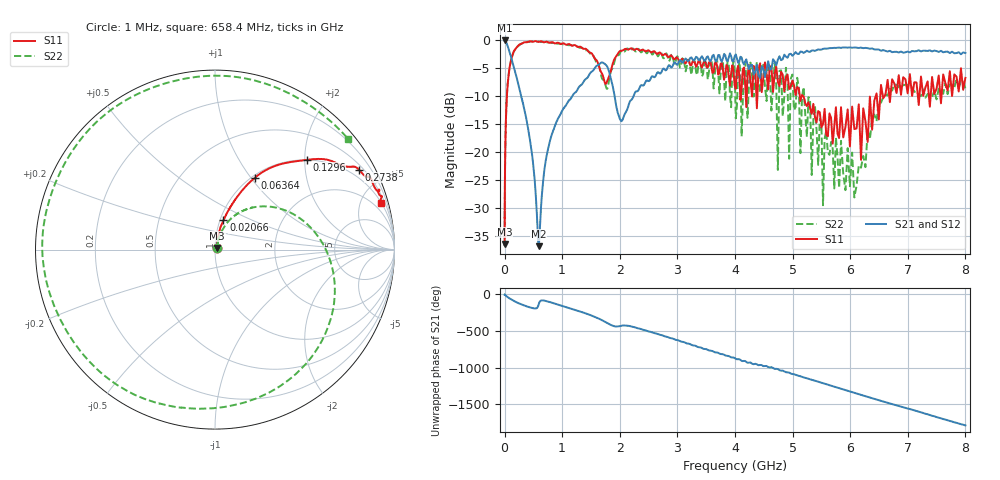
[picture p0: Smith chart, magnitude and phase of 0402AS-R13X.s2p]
!s-Parameter Generated by FASTRON Sdn. Bhd.
!FASTRON P/N : 0402AS-R13X
!Keysight Technologies: E5071C_MY46733604_B.14.02
!Date: Mon Dec 01 10:49:10 2025
!Version  :Rev00  Mon Dec 01 10:49:10 2025
!Data & Calibration Information:
!Freq  S11:SOLT2(ON)  S21:SOLT2(ON)  S12:SOLT2(ON)  S22:SOLT2(ON)
!PortZ  Port1:50+j0  Port2:50+j0
!When reading reference impedance value at option line is always used.
! Remarks : This data is being provided solely for informational purposes.
# Hz S dB R 50
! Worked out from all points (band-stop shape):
!   1601 points, 1 MHz to 8 GHz, reference 50 ohm
!   highest |S21| = -0.09 dB at 2.224 MHz (marker M1); lowest = -36.8 dB at 590.5 MHz (marker M2)
!   |S21| within 3 dB of the highest: start of sweep to 114.4 MHz; 4.916 GHz to end of sweep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
!   lowest |S11| = -36.4 dB at 1.013 MHz (marker M3), VSWR 1.03, Z = 51.2 + j0.899 ohm
!   |S11| at or under -10 dB: start of sweep to 40.56 MHz; 4.092149 GHz to 4.102223 GHz (10.07 MHz wide, 0.246 % of centre); 5.182 GHz to 6.444 GHz (1.262 GHz wide, 21.7 % of centre)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
!   |S22| runs from -36.7 to -0.3 dB; largest |S21 - S12| = 0.015
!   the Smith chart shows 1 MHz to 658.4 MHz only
!   S11 on the Smith chart (normalised r, x): 1 MHz: 1.02, +0.02; 20.66 MHz: 1.04, +0.35; 63.64 MHz: 1.03, +1.05; 129.6 MHz: 1.00, +2.04; 273.8 MHz: 0.67, +3.74; 658.4 MHz: 0.97, +7.08
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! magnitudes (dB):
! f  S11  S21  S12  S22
! 1 MHz  -36.3  -0.1  -0.1  -36.1
! 1.013 MHz  -36.4  -0.1  -0.1  -36.5
! 2.224 MHz  -32.8  -0.1  -0.1  -32.6
! 4.479 MHz  -28.0  -0.1  -0.1  -27.9
! 20.07 MHz  -15.7  -0.3  -0.3  -15.6
! 20.66 MHz  -15.4  -0.3  -0.3  -15.4
! 63.64 MHz  -6.8  -1.4  -1.4  -6.8
! 89.95 MHz  -4.8  -2.2  -2.2  -4.8
! 129.6 MHz  -2.9  -3.7  -3.7  -2.9
! 273.8 MHz  -0.8  -9.4  -9.4  -0.8
! 400.7 MHz  -0.4  -15.4  -15.3  -0.3
! 502 MHz  -0.3  -22.7  -22.6  -0.3
! 590.5 MHz  -0.3  -36.8  -36.8  -0.3
! 658.4 MHz  -0.3  -26.4  -26.4  -0.3
! 901.2 MHz  -0.5  -14.6  -14.6  -0.6
! 1.795 GHz  -7.0  -5.0  -5.1  -8.3
! 2.04 GHz  -1.9  -14.4  -14.4  -1.8
! 3.062 GHz  -3.6  -3.7  -3.7  -4.6
! 4.493 GHz  -6.7  -5.1  -5.1  -4.4
! 5.957 GHz  -12.4  -1.4  -1.4  -19.3
! 6.805 GHz  -9.5  -2.1  -2.1  -8.0
! 8 GHz  -6.8  -2.3  -2.3  -8.7
